FUNCTION_BLOCK FB_DirectoryCopy
(*SwenChen 2011.4.13 ±à¼­*)
VAR_INPUT
	srcNetId				: T_AmsNetId;	(* TwinCAT network address of the source file *)
	srcPathName			: T_MaxString;	(* source file path *)(*Ô´µÄµØÖ·*)
	destNetId			: T_AmsNetId;	(* TwinCAT network address of the destination file *)
	destPathName		: T_MaxString;  	(* destination file path  *)(*Ä¿±êµÄÉÏ²ãµØÖ·*)
	DirectoryName		: T_MaxString;  	(* destination file  name *)(*Ä¿±êÎÄ¼þ¼ÐÃû×Ö*)
	FileType				: STRING;  		(* destination file  name *)(*ÎÄ¼þÀàÐÍ*)
	bExecute			: BOOL;			(* rising edge start fb execution *)
	bFindFileList			: BOOL;			(* rising edge start fb execution *)
	tAdsTimeOut			: TIME;			(* ads timeout *)
	bContinueWhenErr	:BOOL;
	bCancelWhenErr		:BOOL;
END_VAR
VAR_OUTPUT
	bBusy				:BOOL;
	bError				:BOOL;
	nErrId				:UDINT;
	(*==============
	ErrId:=1;		(*ErrId: no find source dir*)
	ErrId:=2;		(*ErrId: no find target dir*)
	ErrId:=3:		target have same file;
	ErrId:=4:		(*Input parameter error*)
	================*)
END_VAR
VAR
	Step				:DWORD;
	RisingEdge			:R_TRIG;
	fbFindFileList:			FB_EnumFindFileList;
	fbEnumFindFileEntry:	FB_EnumFindFileEntry;
	srcFilesLists:			 ARRAY[1..cnMaxRecepeNum]  OF ST_FindFileEntry;
	destFilesLists:		 ARRAY[1..cnMaxRecepeNum]  OF ST_FindFileEntry;
	fbFileCopy:			FB_FileCopy;
	fbCreateDir:			FB_CreateDir;
	i: 					INT;
	n:					INT;
	bFindFileListState		: BOOL;
	TimeCount:			 INT;
END_VAR

RisingEdge(CLK:=bExecute OR bFindFileList);

IF bBusy THEN
	TimeCount:=TimeCount+1;
END_IF

CASE Step OF
	0:	(* do nothing *)
		IF RisingEdge.Q  AND NOT bBusy THEN
			IF bFindFileList THEN
				bFindFileListState:=TRUE;
				bBusy := TRUE;
				Step := 40;
			ELSE
				bFindFileListState:=FALSE;
				IF DirectoryName=''
				OR FileType=''
				OR srcPathName=''
				OR destPathName='' THEN		(*Input parameter error*)
					bError:=TRUE;
					nErrId:=4;
				ELSE
					bBusy := TRUE;
					bError:= FALSE;
					TimeCount:=0;
					nErrId:=0;
					Step := 10;
				END_IF
			END_IF
		END_IF

	10:	(* find source dir*)
		fbEnumFindFileEntry
			(
			sNetId:='' , 
			sPathName:=CONCAT(srcPathName,DirectoryName),
			eCmd:=eEnumCmd_First ,
			bExecute:=TRUE ,
			tTimeout:=T#10s ,
			);
		IF NOT  fbEnumFindFileEntry.bBusy THEN
			IF NOT  fbEnumFindFileEntry.bEOE THEN		(*target dir is exist*)
				Step := 20;
			ELSE										(*target dir no exist*)
				bError:=TRUE;
				nErrId:=1;		(*ErrId: no find source dir*)
				Step:=70;
			END_IF
			fbEnumFindFileEntry(bExecute:=FALSE);
		END_IF

	11:	(*Wait*)
		IF bContinueWhenErr OR bCancelWhenErr THEN
			bError:=FALSE;
			nErrId:=0;
			Step:=0;
		END_IF

	20:	(*find Target Dir*)
		fbEnumFindFileEntry
			(
			sNetId:='' , 
			sPathName:=CONCAT(destPathName,DirectoryName),
			eCmd:=eEnumCmd_First ,
			bExecute:=TRUE ,
			tTimeout:=T#10s ,
			);
		IF NOT  fbEnumFindFileEntry.bBusy THEN
			IF NOT  fbEnumFindFileEntry.bEOE THEN	(*target dir is exist*)
				Step := 40;
			ELSE									(*target dir no exist*)
				Step:=30;
			END_IF
			fbEnumFindFileEntry(bExecute:=FALSE);
		END_IF

	30:	(*createt dir  *)
		fbCreateDir
			(
			sNetId:='',
			sPathName:= CONCAT(destPathName,DirectoryName),
			ePath:= PATH_GENERIC,
			bExecute:=TRUE,
			tTimeout:=t#10s
			);
		IF NOT fbCreateDir.bBusy THEN
			fbCreateDir(bExecute:=FALSE);
			Step:=40;
		END_IF

	40:	(*Find source FileList*)
		fbFindFileList
			(
			sNetID:='',
			sPathName:=CONCAT(CONCAT(CONCAT(srcPathName,DirectoryName),'\*.'),FileType),
			eCmd:= eEnumCmd_First,
			pFindList:= ADR(srcFilesLists),
			cbFindList:=SIZEOF(srcFilesLists),
			bExecute:= TRUE ,
			tTimeout:=t#10s
			);
		IF NOT fbFindFileList.bBusy THEN
			fbFindFileList(bExecute:=FALSE);
			IF bFindFileList OR bFindFileListState THEN
				Step:=70;
			ELSE
				Step:=41;
			END_IF
		END_IF

	41:	(*Find target FileList*)
		fbFindFileList
			(
			sNetID:='',
			sPathName:=CONCAT(CONCAT(CONCAT(destPathName,DirectoryName),'\*.'),FileType),
			eCmd:= eEnumCmd_First,
			pFindList:= ADR(destFilesLists),
			cbFindList:=SIZEOF(destFilesLists),
			bExecute:= TRUE ,
			tTimeout:=t#10s
			);
		IF NOT fbFindFileList.bBusy THEN
			fbFindFileList(bExecute:=FALSE);
			Step:=50;
			i:=1;
		END_IF


	50:	(*check no same mane file*)
		IF srcFilesLists[i].sFileName='' THEN
			IF i>=15 THEN
				i:=1;
				Step:=70;
			ELSE
				i:=i+1;
			END_IF
		ELSE
			FOR n:=1 TO 15 DO
				IF destFilesLists[n].sFileName =  srcFilesLists[i].sFileName THEN
					bError:=TRUE;
					nErrId:=3;
				END_IF
			END_FOR
			IF  bError THEN			(*if exiest same file *)
				IF bContinueWhenErr THEN
					Step:=60;
					bError:=FALSE;
					nErrId:=0;
				ELSIF bCancelWhenErr THEN
					i:=i+1;
					bError:=FALSE;
					nErrId:=0;
				END_IF
			ELSE					(*no same file *)
				fbFileCopy
					(
					srcNetId:='' ,
					srcFileName:=CONCAT(CONCAT(CONCAT(srcPathName,DirectoryName),'\'),srcFilesLists[i].sFileName) ,
					cbReadLen:=srcFilesLists[i].fileSize.dwLowPart,
					destNetId:='' ,
					destFileName:=CONCAT(CONCAT(CONCAT(destPathName,DirectoryName),'\'),srcFilesLists[i].sFileName) ,
					bExecute:=TRUE ,
					tAdsTimeOut:=T#10s ,
					);
				Step:=60;
			END_IF
		END_IF

	60:	(*copy*)
		fbFileCopy();
		IF NOT fbFileCopy.bBusy THEN
			fbFileCopy(bExecute:=FALSE);
			IF i>=15 THEN
				i:=1;
				Step:=70;
			ELSE
				i:=i+1;
				Step:=50;
			END_IF
		END_IF

	70:	(*finish*)
		bFindFileListState:=FALSE;
		bBusy := FALSE;
		Step:=0;

END_CASE

END_FUNCTION_BLOCK
